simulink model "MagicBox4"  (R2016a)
settings: Solver=VariableStepAuto  StartTime=0.0  StopTime=inf  RelTol=1e-3
libraries: simulink x1

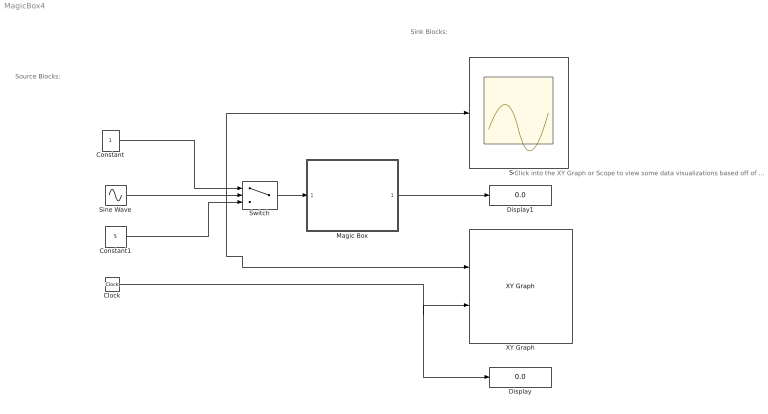
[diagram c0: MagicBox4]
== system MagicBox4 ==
  note: Click into the XY Graph or Scope to view some data visualizations based off of the source blocks
  note: Sink Blocks:
  note: Source Blocks:
  Clock : Clock
  Constant : Constant
  Constant1 : Constant  Value=5
  Display : Display
  Display1 : Display
  Magic Box : MATLAB Function  TreatAsAtomicUnit=on
  Scope : Scope
  Sine Wave : Sin  SampleTime=0
  Switch : Switch  Criteria=u2 > Threshold
  XY Graph : simulink/Sinks/XY Graph  xmin=-1  xmax=1  ymin=-1  ymax=1  st=-1
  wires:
  Constant/1 -> Switch/1
  Magic Box/1(output) -> Display1/1
  Constant1/1 -> Switch/3
  Switch/1 -> Magic Box/1(input)
  Sine Wave/1 -> XY Graph/1, Scope/1, Switch/2
  Clock/1 -> XY Graph/2, Display/1

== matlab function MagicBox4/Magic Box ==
function output = MagicBox(input)
number = input;
output = number+1;
end
